ORGANIZATION_BLOCK OB 1
BEGIN

	// Check instance-DB length
	AUF		DB 1
	L		DBLG
	__ASSERT==	__ACCU 1,	22
	AUF		DB 0

BE //TODO

	// Check TON
	CALL	SFB 4, DB 1 (
		IN	:= FALSE,
		PT	:= T#0S,
		Q	:= M 0.0,
		ET	:= MD 2,
	)
	U		M 0.0
	__ASSERT==	__STW VKE,	0
	L		MD 2
	__ASSERT==	__ACCU 1,	0
	L		DB1.DBB 12	// STATE
	__ASSERT==	__ACCU 1,	0
	L		DB1.DBD 14	// STIME
	__ASSERT==	__ACCU 1,	0
	L		DB1.DBD 18	// ATIME
	__ASSERT>=	__ACCU 1,	__ACCU 2

	CALL	SFB 4, DB 1 (
		IN	:= FALSE,
		PT	:= T#100MS,
		Q	:= M 0.0,
		ET	:= MD 2,
	)
	U		M 0.0
	__ASSERT==	__STW VKE,	0
	L		MD 2
	__ASSERT==	__ACCU 1,	0
	L		DB1.DBB 12	// STATE
	__ASSERT==	__ACCU 1,	0
	L		DB1.DBD 14	// STIME
	__ASSERT==	__ACCU 1,	0
	L		DB1.DBD 18	// ATIME
	__ASSERT>=	__ACCU 1,	__ACCU 2



END_ORGANIZATION_BLOCK


DATA_BLOCK DB 1
	SFB 4
BEGIN
END_DATA_BLOCK
